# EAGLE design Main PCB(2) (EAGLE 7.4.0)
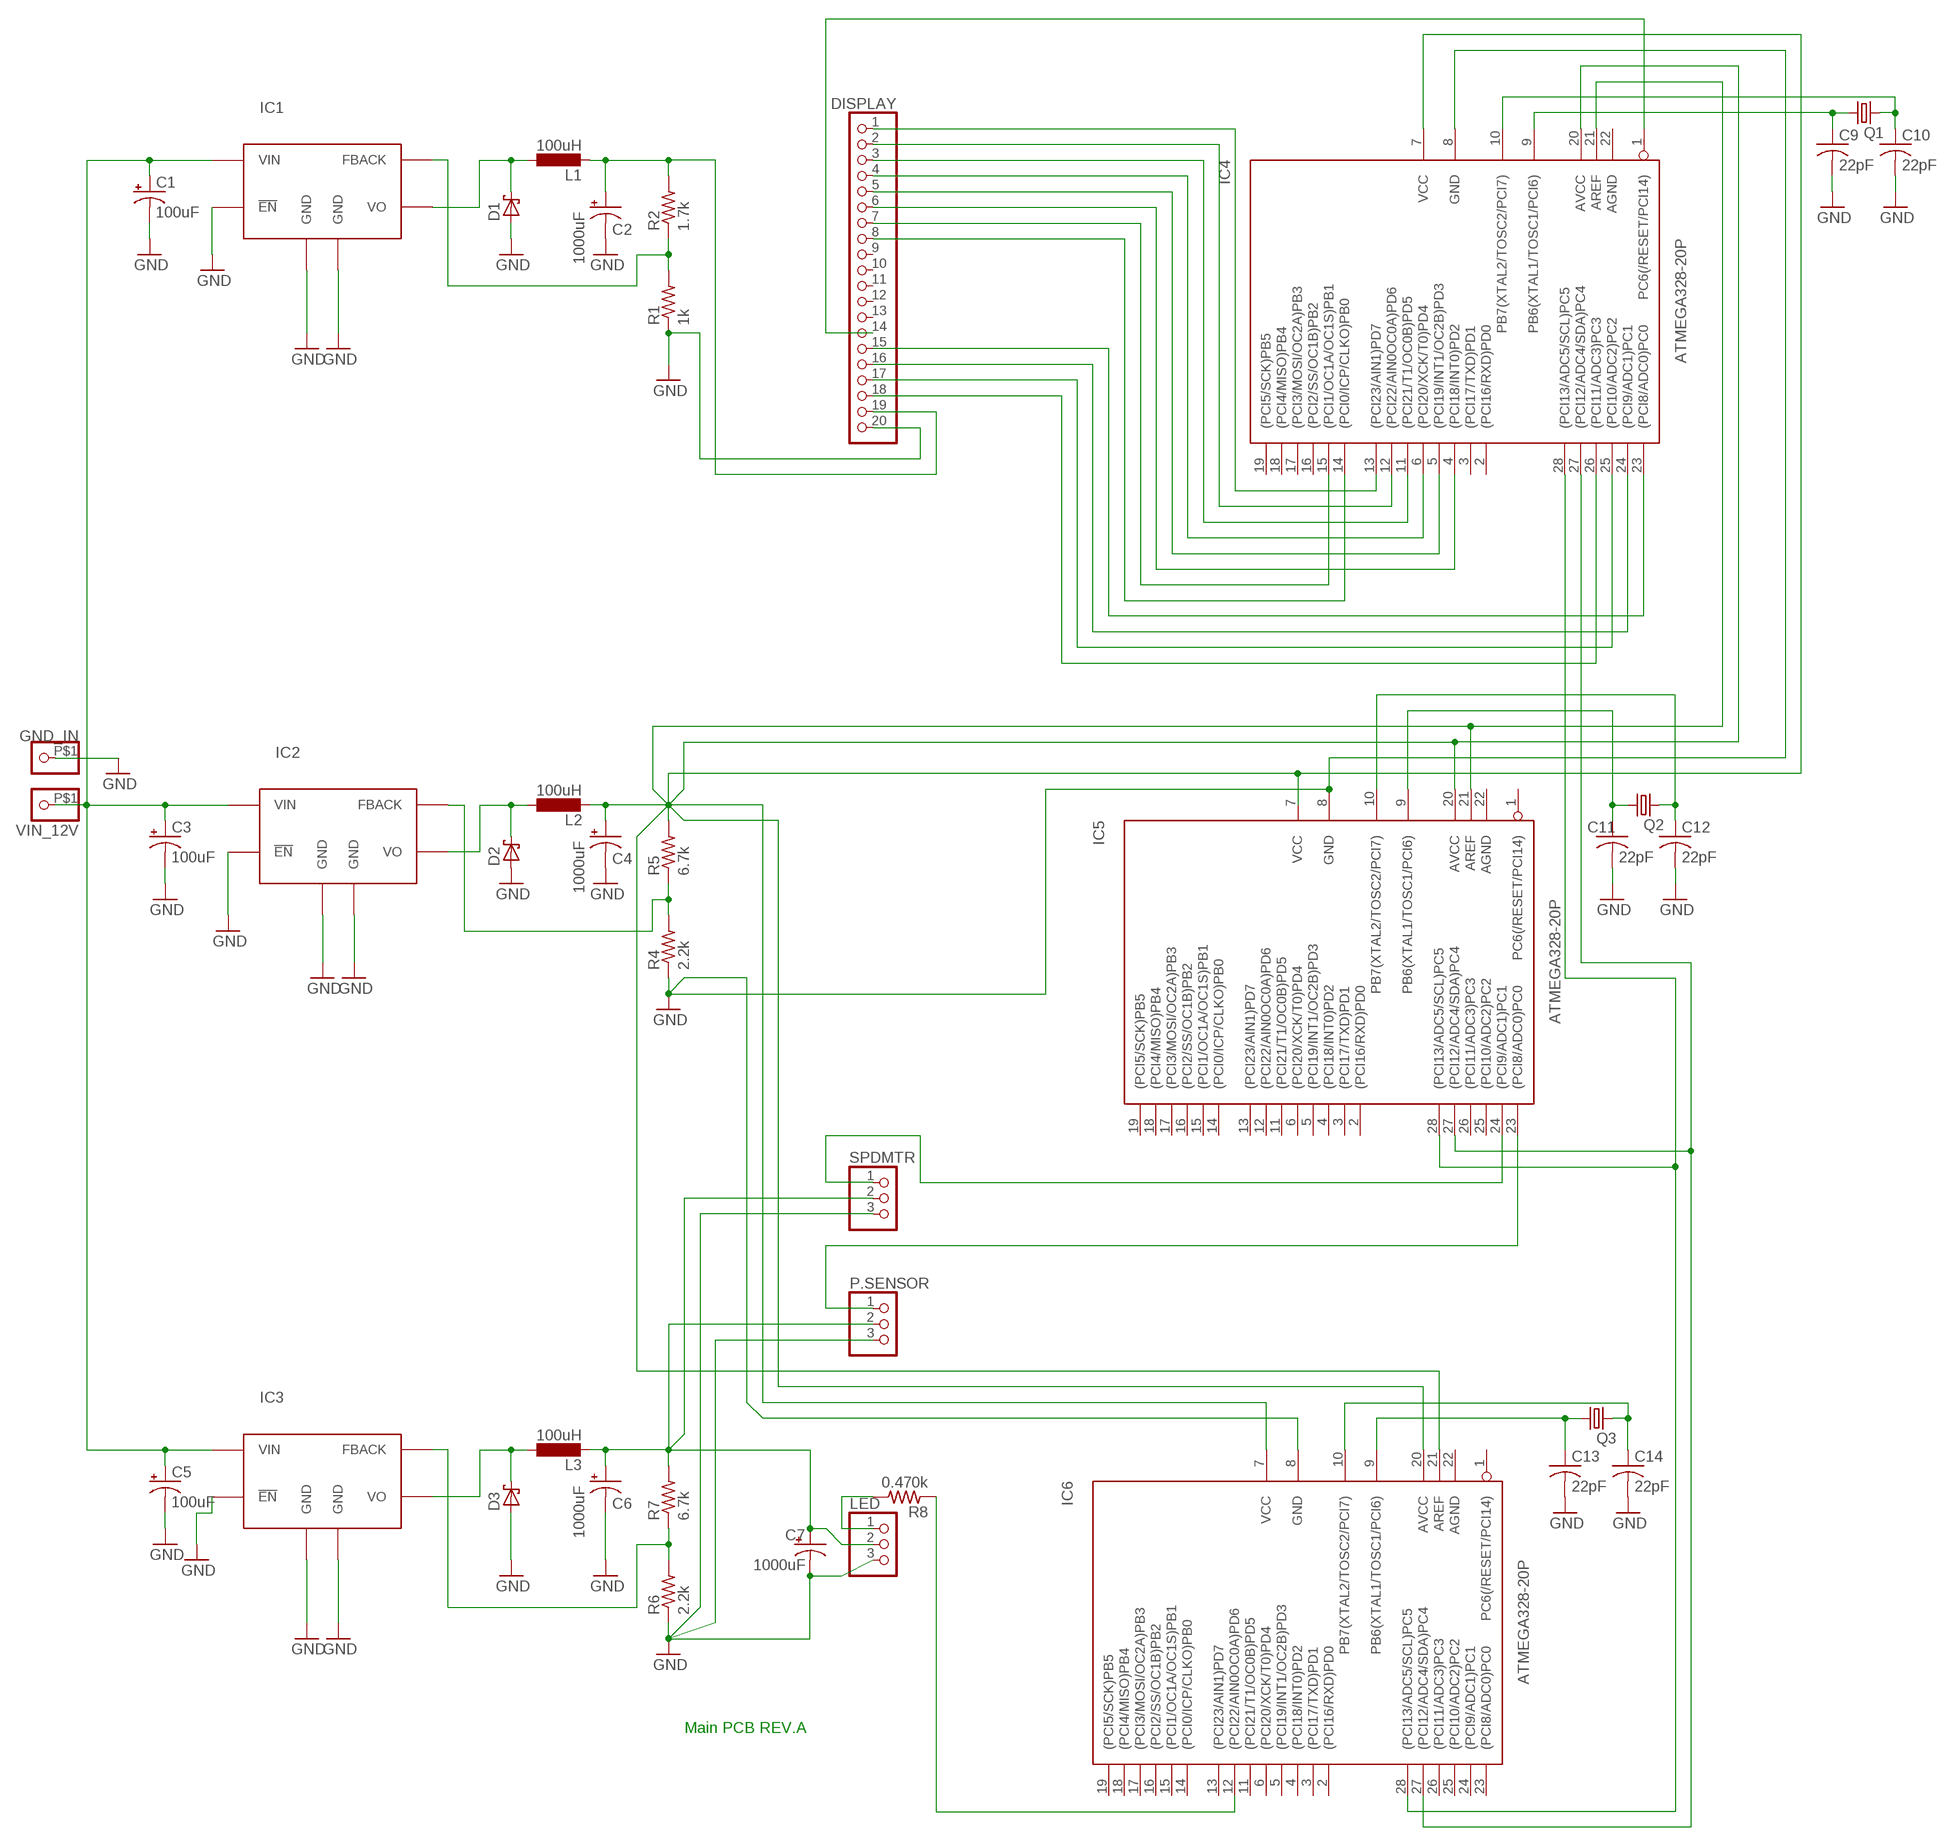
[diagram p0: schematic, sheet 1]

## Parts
C1  100uF  CAP_POLPTH1  [CPOL-RADIAL-100UF-25V]
C2  1000uF  CAP_POLPTH4  [CPOL-RADIAL-1000UF-25V]
C3  100uF  CAP_POLPTH1  [CPOL-RADIAL-100UF-25V]
C4  1000uF  CAP_POLPTH4  [CPOL-RADIAL-1000UF-25V]
C5  100uF  CAP_POLPTH1  [CPOL-RADIAL-100UF-25V]
C6  1000uF  CAP_POLPTH4  [CPOL-RADIAL-1000UF-25V]
C7  1000uF  CAP_POLPTH4  [CPOL-RADIAL-1000UF-25V]
C9  22pF  C-US025-024X044  [C025-024X044]
C10  22pF  C-US025-024X044  [C025-024X044]
C11  22pF  C-US025-024X044  [C025-024X044]
C12  22pF  C-US025-024X044  [C025-024X044]
C13  22pF  C-US025-024X044  [C025-024X044]
C14  22pF  C-US025-024X044  [C025-024X044]
D1  BYV10  [DO41-10]
D2  BYV10  [DO41-10]
D3  BYV10  [DO41-10]
DISPLAY  PINHD-1X20  [1X20]
GND_IN  PINHD-1X1-BIGPOGO  [1X1-BIGPOGO]
IC1  LM2576S  [TO263-5]
IC2  LM2576S  [TO263-5]
IC3  LM2576S  [TO263-5]
IC4  ATMEGA328-20P  [DIL28-3]
IC5  ATMEGA328-20P  [DIL28-3]
IC6  ATMEGA328-20P  [DIL28-3]
L1  100uH  L-EUTJ3-U2  [TJ3-U2]
L2  100uH  L-EUTJ3-U2  [TJ3-U2]
L3  100uH  L-EUTJ3-U2  [TJ3-U2]
LED  PINHD-1X3  [1X03]
P.SENSOR  PINHD-1X3  [1X03]
Q1  CRYSTALTC26V  [TC26V]
Q2  CRYSTALTC26V  [TC26V]
Q3  CRYSTALTC26V  [TC26V]
R1  1k  R-US_0204/5  [0204/5]
R2  1.7k  R-US_0204/5  [0204/5]
R4  2.2k  R-US_0204/5  [0204/5]
R5  6.7k  R-US_0204/5  [0204/5]
R6  2.2k  R-US_0204/5  [0204/5]
R7  6.7k  R-US_0204/5  [0204/5]
R8  0.470k  R-US_0204/5  [0204/5]
SPDMTR  PINHD-1X3  [1X03]
VIN_12V  PINHD-1X1-BIGPOGO  [1X1-BIGPOGO]

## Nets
GND [Supply]: C1.2(-) C2.- C3.2(-) C4.- C5.2(-) C6.- C7.- C9.2 C10.2 C11.2 C12.2 C13.2 C14.2 D1.A D2.A D3.A DISPLAY.20 GND_IN.P$1 IC1.3(GND) IC1.5(!EN) IC1.TAB(GND) IC2.3(GND) IC2.5(!EN) IC2.TAB(GND) IC3.3(GND) IC3.5(!EN) IC3.TAB(GND) IC4.8(GND) IC5.8(GND) IC6.8(GND) LED.3 P.SENSOR.3 R1.1 R4.1 R6.1 SPDMTR.3
LED: IC4.27((PCI12/ADC4/SDA)PC4) IC5.27((PCI12/ADC4/SDA)PC4) IC6.27((PCI12/ADC4/SDA)PC4)
N$1 [Supply]: C1.1(+) C3.1(+) C5.1(+) IC1.1(VIN) IC2.1(VIN) IC3.1(VIN) VIN_12V.P$1
N$2 [Supply]: D1.C IC1.2(VO) L1.1
N$3 [Supply]: D3.C IC3.2(VO) L3.1
N$4: LED.1 R8.2
N$5 [Supply]: IC3.4(FBACK) R6.2 R7.1
N$6: DISPLAY.18 IC4.26((PCI11/ADC3)PC3)
N$7: C12.1 IC5.10(PB7(XTAL2/TOSC2/PCI7)) Q2.2
N$8 [Supply]: IC2.4(FBACK) R4.2 R5.1
N$10: DISPLAY.1 IC4.13((PCI23/AIN1)PD7)
N$11: IC5.24((PCI9/ADC1)PC1) SPDMTR.1
N$12 [Supply]: D2.C IC2.2(VO) L2.1
N$13: IC4.28((PCI13/ADC5/SCL)PC5) IC5.28((PCI13/ADC5/SCL)PC5) IC6.28((PCI13/ADC5/SCL)PC5)
N$14: IC6.12((PCI22/AIN0OC0A)PD6) R8.1
N$15: DISPLAY.2 IC4.12((PCI22/AIN0OC0A)PD6)
N$16: DISPLAY.3 IC4.11((PCI21/T1/OC0B)PD5)
N$17: DISPLAY.4 IC4.6((PCI20/XCK/T0)PD4)
N$18 [Supply]: C4.+ IC4.7(VCC) IC4.20(AVCC) IC4.21(AREF) IC5.20(AVCC) IC5.21(AREF) IC6.7(VCC) IC6.20(AVCC) IC6.21(AREF) L2.2 R5.2
N$19: C11.1 IC5.9(PB6(XTAL1/TOSC1/PCI6)) Q2.1
N$20: C14.1 IC6.10(PB7(XTAL2/TOSC2/PCI7)) Q3.2
N$21: DISPLAY.15 IC4.23((PCI8/ADC0)PC0)
N$22 [Supply]: C2.+ DISPLAY.19 L1.2 R2.2
N$23: IC5.23((PCI8/ADC0)PC0) P.SENSOR.1
N$24: DISPLAY.16 IC4.24((PCI9/ADC1)PC1)
N$25: DISPLAY.17 IC4.25((PCI10/ADC2)PC2)
N$26: DISPLAY.5 IC4.5((PCI19/INT1/OC2B)PD3)
N$27: DISPLAY.6 IC4.4((PCI18/INT0)PD2)
N$28: C13.1 IC6.9(PB6(XTAL1/TOSC1/PCI6)) Q3.1
N$29: DISPLAY.7 IC4.15((PCI1/OC1A/OC1S)PB1)
N$30: DISPLAY.8 IC4.14((PCI0/ICP/CLKO)PB0)
N$31: DISPLAY.14 IC4.1(PC6(/RESET/PCI14))
N$32 [Supply]: C6.+ C7.+ L3.2 LED.2 P.SENSOR.2 R7.2 SPDMTR.2
N$33: C10.1 IC4.10(PB7(XTAL2/TOSC2/PCI7)) Q1.2
N$34: C9.1 IC4.9(PB6(XTAL1/TOSC1/PCI6)) Q1.1
N$38 [Supply]: IC1.4(FBACK) R1.2 R2.1
Unconnected: DISPLAY.9 DISPLAY.10 DISPLAY.11 DISPLAY.12 DISPLAY.13 IC4.2((PCI16/RXD)PD0) IC4.3((PCI17/TXD)PD1) IC4.16((PCI2/SS/OC1B)PB2) IC4.17((PCI3/MOSI/OC2A)PB3) IC4.18((PCI4/MISO)PB4) IC4.19((PCI5/SCK)PB5) IC4.22(AGND) IC5.1(PC6(/RESET/PCI14)) IC5.2((PCI16/RXD)PD0) IC5.3((PCI17/TXD)PD1) IC5.4((PCI18/INT0)PD2) IC5.5((PCI19/INT1/OC2B)PD3) IC5.6((PCI20/XCK/T0)PD4) IC5.7(VCC) IC5.11((PCI21/T1/OC0B)PD5) IC5.12((PCI22/AIN0OC0A)PD6) IC5.13((PCI23/AIN1)PD7) IC5.14((PCI0/ICP/CLKO)PB0) IC5.15((PCI1/OC1A/OC1S)PB1) IC5.16((PCI2/SS/OC1B)PB2) IC5.17((PCI3/MOSI/OC2A)PB3) IC5.18((PCI4/MISO)PB4) IC5.19((PCI5/SCK)PB5) IC5.22(AGND) IC5.25((PCI10/ADC2)PC2) IC5.26((PCI11/ADC3)PC3) IC6.1(PC6(/RESET/PCI14)) IC6.2((PCI16/RXD)PD0) IC6.3((PCI17/TXD)PD1) IC6.4((PCI18/INT0)PD2) IC6.5((PCI19/INT1/OC2B)PD3) IC6.6((PCI20/XCK/T0)PD4) IC6.11((PCI21/T1/OC0B)PD5) IC6.13((PCI23/AIN1)PD7) IC6.14((PCI0/ICP/CLKO)PB0) IC6.15((PCI1/OC1A/OC1S)PB1) IC6.16((PCI2/SS/OC1B)PB2) IC6.17((PCI3/MOSI/OC2A)PB3) IC6.18((PCI4/MISO)PB4) IC6.19((PCI5/SCK)PB5) IC6.22(AGND) IC6.23((PCI8/ADC0)PC0) IC6.24((PCI9/ADC1)PC1) IC6.25((PCI10/ADC2)PC2) IC6.26((PCI11/ADC3)PC3)

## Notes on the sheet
- Main PCB REV.A

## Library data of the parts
C1 C3 C5 = SparkFun-Capacitors:CAP_POL: Capacitor Polarized; MPN: UPW1E101MED; OC_NEWARK: 55K0210
C2 C4 C6 C7 = SparkFun-Capacitors:CAP_POL: Capacitor Polarized; MF: UNITED CHEMI-CON; MPN: EKMG160ELL102MJ16S; OC_NEWARK: 23K3576
C9-C14 = adafruit:C-US: CAPACITOR, American symbol; MPN: MCCC50V220JNPO; OC_NEWARK: 97M5068
D1-D3 = diode:BYV10: DIODE; MPN: 1N5818-E3/54; OC_NEWARK: 78K2605
DISPLAY = adafruit:PINHD-1X20: PIN HEADER; MF: MILL MAX MFG. CORP.; MPN: 310-93-120-41-001; OC_NEWARK: 66F6053
GND_IN VIN_12V = adafruit:PINHD-1X1: Pin header 1x1 for 0.1" spacing; OC_NEWARK: unknown
IC1-IC3 = AWJLEagleLib:LM2576: Texas Instruments LM2576 Simple Switcher
IC4-IC6 = atmega328:ATMEGA328*P: MICROCONTROLLER 32 kBytes FLASH 2 kBytes SRAM 1 kBytes EEPROM USART 8-channel 10 bit ADC; MPN: A000048; OC_NEWARK: 13T9287
L1-L3 = resistor:L-EU: INDUCTOR, European symbol; MPN: RL622-101K-RC; OC_NEWARK: 86K3359
LED P.SENSOR SPDMTR = adafruit:PINHD-1X3: PIN HEADER; OC_NEWARK: unknown
Q1-Q3 = adafruit:CRYSTAL: CRYSTAL; MF: Abracon Corporation; MPN: ABL-20.000MHZ-B2; OC_FARNELL: unknown; OC_NEWARK: 13J1633
R1 R2 R5 R7 R8 = rcl:R-US_: RESISTOR, American symbol; OC_NEWARK: unknown
R4 R6 = rcl:R-US_: RESISTOR, American symbol; MPN: ERJ-2GEJ620X; OC_NEWARK: 53W4174

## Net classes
0 default: width 0.305 mm, drill 0.508 mm, clearance 0.254 mm
1 Supply: width 1.27 mm, drill 0.508 mm, clearance 0.254 mm to class 0, clearance 0.205 mm

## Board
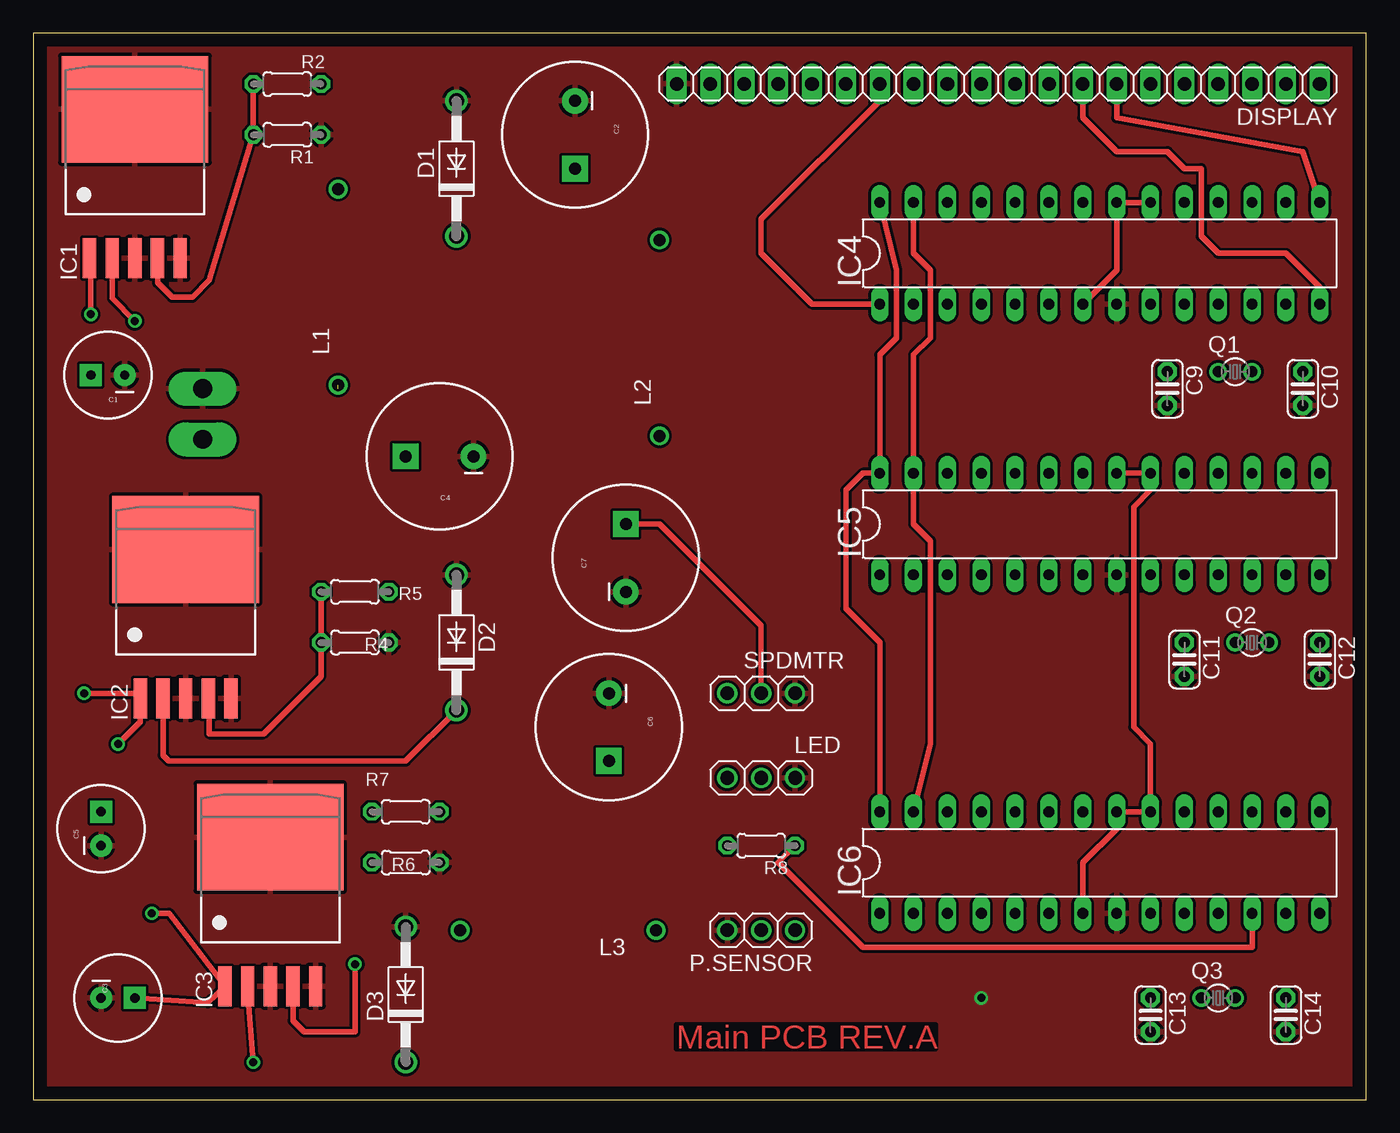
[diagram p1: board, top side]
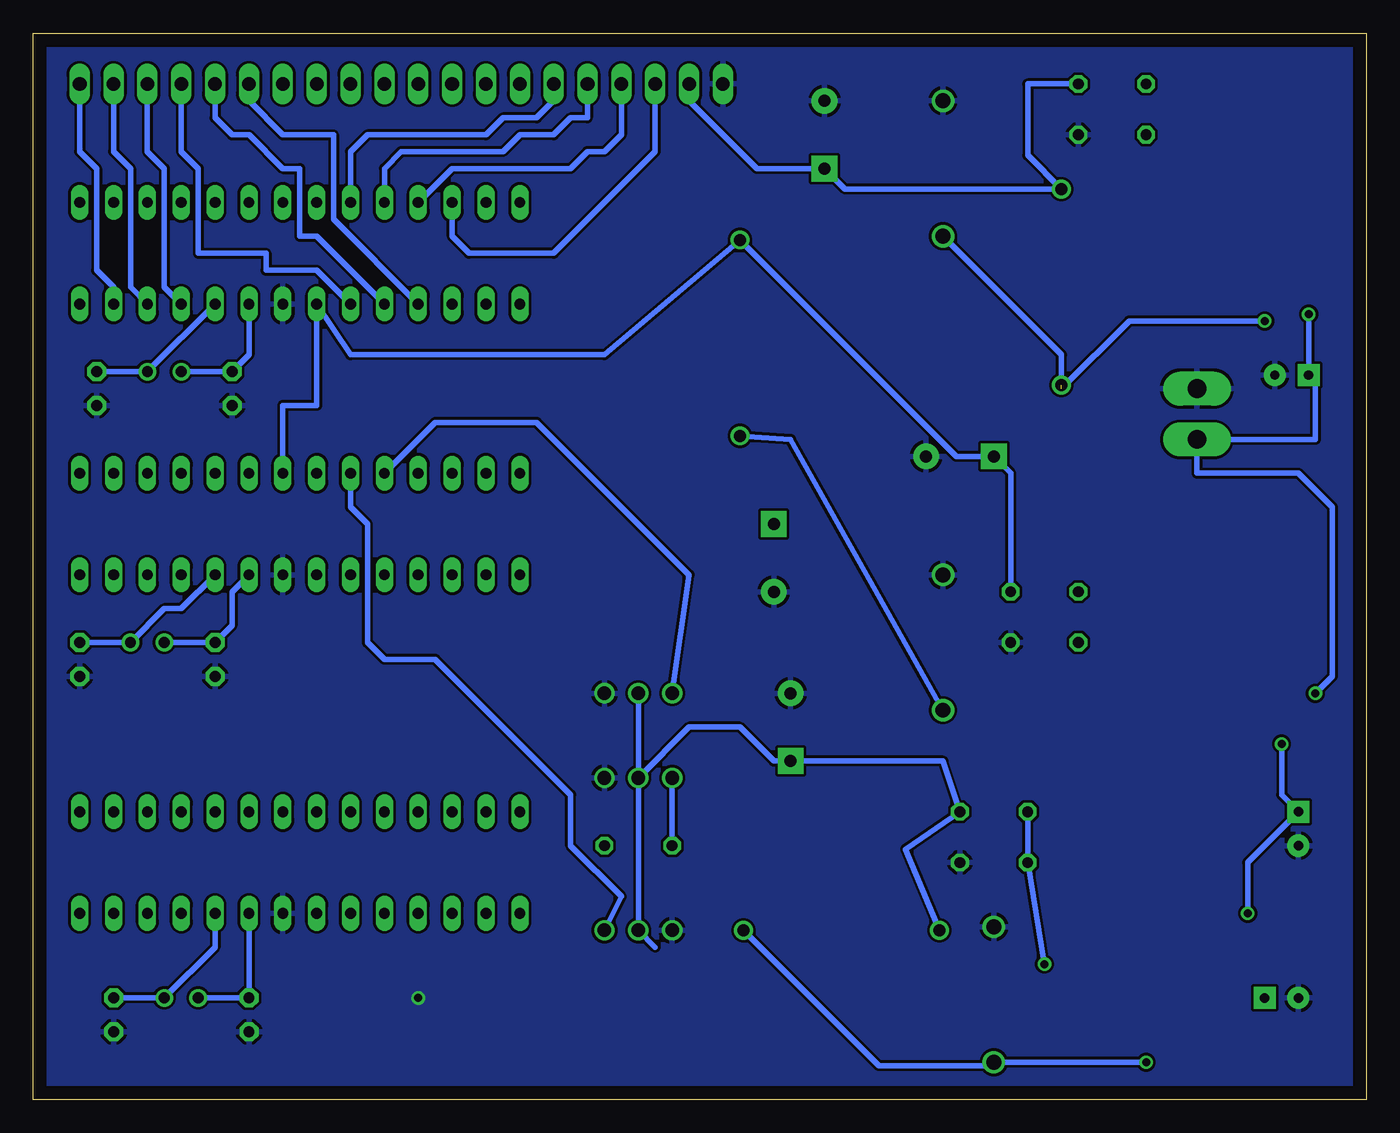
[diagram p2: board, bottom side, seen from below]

Size 100 x 80 mm. Coordinates in mm from the lower left corner, seen from the top.
Outline: 0,0 100,0 100,80 0,80 0,0
Copper layers (1*16): Top 0.035mm / dielectric 1.5mm / Bottom 0.035mm
Design rules "Main PCB(2)": minimum track width 10mil, minimum drill 24mil, track to track 0.205mm, track to pad 0.205mm, pad to pad 0.205mm, via to via 0.205mm, smd to smd 8mil, copper to edge 40mil, drill to drill 8mil, minimum pad ring 10mil, minimum via ring 8mil, stop-mask expansion 4mil, vias tented up to drill 0mil, thermal gap 10mil

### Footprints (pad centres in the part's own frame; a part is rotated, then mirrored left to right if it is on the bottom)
CPOL-RADIAL-100UF-25V = drill 0.7 pad 1.651 square: 1 1.27,0 | drill 0.7 pad 1.651: 2 -1.27,0
CPOL-RADIAL-1000UF-25V = drill 0.9 pad 1.93 square: + 2.54,0 | drill 0.9 pad 1.93: - -2.54,0
C025-024X044 = drill 0.813 pad 1.422 octagon: 1 -1.27,0; 2 1.27,0
DO41-10 = drill 1.118: A 5.08,0; C -5.08,0
1X20 = drill 1.016 long: 1 -24.13,0; 2 -21.59,0; 3 -19.05,0; 4 -16.51,0; 5 -13.97,0; 6 -11.43,0; 7 -8.89,0; 8 -6.35,0; 9 -3.81,0; 10 -1.27,0; 11 1.27,0; 12 3.81,0; 13 6.35,0; 14 8.89,0; 15 11.43,0; 16 13.97,0; 17 16.51,0; 18 19.05,0; 19 21.59,0; 20 24.13,0
1X1-BIGPOGO = drill 1.4 pad 2.54 long: P$1 0,0
TO263-5 = smd 1 x 3: 1 -3.4,-8; 2 -1.7,-8; 3 0,-8; 4 1.7,-8; 5 3.4,-8 | smd 11 x 8: TAB 0,3.175
DIL28-3 = drill 0.813 long: 1 -16.51,-3.81; 2 -13.97,-3.81; 3 -11.43,-3.81; 4 -8.89,-3.81; 5 -6.35,-3.81; 6 -3.81,-3.81; 7 -1.27,-3.81; 8 1.27,-3.81; 9 3.81,-3.81; 10 6.35,-3.81; 11 8.89,-3.81; 12 11.43,-3.81; 13 13.97,-3.81; 14 16.51,-3.81; 15 16.51,3.81; 16 13.97,3.81; 17 11.43,3.81; 18 8.89,3.81; 19 6.35,3.81; 20 3.81,3.81; 21 1.27,3.81; 22 -1.27,3.81; 23 -3.81,3.81; 24 -6.35,3.81; 25 -8.89,3.81; 26 -11.43,3.81; 27 -13.97,3.81; 28 -16.51,3.81
TJ3-U2 = drill 0.9: 1 -7.35,0; 2 7.35,0
1X03 = drill 1.016: 1 -2.54,0; 2 0,0; 3 2.54,0
TC26V = drill 0.813: 1 -1.27,0; 2 1.27,0
0204/5 = drill 0.813 octagon: 1 -2.54,0; 2 2.54,0

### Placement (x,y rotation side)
C1  5.59,54.36 180 top
C2  40.64,72.39 270 top
C3  6.35,7.62 0 top
C4  30.48,48.26 180 top
C5  5.08,20.32 90 top
C6  43.18,27.94 270 top
C7  44.45,40.64 90 top
C9  85.09,53.34 270 top
C10  95.25,53.34 270 top
C11  86.36,33.02 270 top
C12  96.52,33.02 270 top
C13  83.82,6.35 270 top
C14  93.98,6.35 270 top
D1  31.75,69.85 90 top
D2  31.75,34.29 90 top
D3  27.94,7.87 90 top
DISPLAY  72.39,76.2 180 top
GND_IN  12.7,53.34 0 top
IC1  7.62,71.12 0 top
IC2  11.43,38.1 0 top
IC3  17.78,16.51 0 top
IC4  80.01,63.5 0 top
IC5  80.01,43.18 0 top
IC6  80.01,17.78 0 top
L1  22.86,60.96 90 top
L2  46.99,57.15 90 top
L3  39.37,12.7 180 top
LED  54.61,24.13 0 top
P.SENSOR  54.61,12.7 180 top
Q1  90.17,54.61 0 top
Q2  91.44,34.29 0 top
Q3  88.9,7.62 0 top
R1  19.05,72.39 180 top
R2  19.05,76.2 0 top
R4  24.13,34.29 180 top
R5  24.13,38.1 0 top
R6  27.94,17.78 180 top
R7  27.94,21.59 0 top
R8  54.61,19.05 180 top
SPDMTR  54.61,30.48 0 top
VIN_12V  12.7,49.53 0 top

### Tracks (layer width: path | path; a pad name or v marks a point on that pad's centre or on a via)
GND  (via drill 0.6)
  other vias: 71.12,7.62
  pour Top: -1.27,81.28 -1.27,-1.27 101.6,-1.27 101.6,81.28
  pour Bottom: -2.54,82.55 -2.54,-2.54 102.87,-2.54 102.87,-1.27 102.87,82.55
LED
  Top 0.406: IC4.27 66.04,63.5 67.31,62.23 67.31,57.15 66.04,55.88 IC5.27 66.04,43.18 67.31,41.91 67.31,26.67 IC6.27
N$1  (via drill 0.6)
  Top 0.406: IC1.1 4.32,63.12 v4.32,58.93 | v3.81,30.48 7.65,30.48 IC2.1 8.03,28.35 v6.35,26.67 | v8.89,13.97 10.19,13.97 IC3.1 13.08,7.24 C3.1
  Bottom 0.406: v4.32,58.93 C1.1 3.81,54.36 3.81,49.53 VIN_12V.P$1 12.7,46.99 5.08,46.99 2.54,44.45 2.54,31.75 v3.81,30.48 | v6.35,26.67 6.35,22.86 C5.1 8.89,17.78 v8.89,13.97
N$2  (via drill 0.6)  (1 unrouted)
  Top 0.406: IC1.2 5.92,60.12 v7.62,58.42
  Bottom 0.406: v7.62,58.42 17.78,58.42 22.86,53.34 | L1.1 22.86,55.88 D1.C
N$3  (via drill 0.6)
  Top 0.406: IC3.2 16.08,8.05 v16.51,2.79
  Bottom 0.406: v16.51,2.79 D3.C 27.94,2.54 36.56,2.54 L3.1
N$4
  Bottom 0.406: LED.1 R8.2
N$5  (via drill 0.6)
  Top 0.406: IC3.4 19.48,5.92 20.32,5.08 24.13,5.08 v24.13,10.16
  Bottom 0.406: v24.13,10.16 R6.2 R7.1
N$6
  Bottom 0.406: DISPLAY.18 53.34,71.12 60.96,63.5 67.31,63.5 68.58,64.77 IC4.26
N$7
  Bottom 0.406: IC5.10 88.9,36.83 90.17,36.83 Q2.2 C12.1
N$8
  Top 0.406: IC2.4 13.21,30.1 13.21,27.43 17.27,27.43 21.59,31.75 R4.2 R5.1
N$10
  Bottom 0.406: DISPLAY.1 96.52,71.12 95.25,69.85 95.25,62.23 93.98,60.96 IC4.13
N$11
  Bottom 0.406: SPDMTR.1 50.8,39.37 62.23,50.8 69.85,50.8 IC5.24
N$12
  Top 0.406: IC2.2 9.73,25.83 10.16,25.4 27.94,25.4 D2.C
  Bottom 0.406: D2.C 43.18,49.53 L2.1
N$13
  Top 0.406: IC6.28 63.5,34.29 60.96,36.83 60.96,45.72 62.23,46.99 IC5.28 63.5,55.88 64.77,57.15 64.77,62.23 IC4.28
N$14
  Top 0.406: R8.1 55.88,17.78 62.23,11.43 91.44,11.43 IC6.12
N$15
  Bottom 0.406: DISPLAY.2 93.98,71.12 92.71,69.85 92.71,60.96 IC4.12
N$16
  Bottom 0.406: DISPLAY.3 91.44,71.12 90.17,69.85 90.17,60.96 IC4.11
N$17
  Bottom 0.406: DISPLAY.4 88.9,71.12 87.63,69.85 87.63,63.5 82.55,63.5 82.55,62.23 78.74,62.23 IC4.6
N$18
  Top 0.406: IC5.21 IC5.20 83.82,45.72 82.55,44.45 82.55,27.94 83.82,26.67 IC6.20 IC6.21 81.28,20.32 78.74,17.78 IC6.7 | IC4.20 IC4.21 81.28,62.23 IC4.7
  Bottom 0.406: IC5.21 81.28,52.07 78.74,52.07 IC4.7 76.2,55.88 57.15,55.88 L2.2 30.75,48.26 C4.+ 26.67,46.99 R5.2
N$19
  Bottom 0.406: IC5.9 85.09,38.1 85.09,35.56 C11.1 Q2.1
N$20
  Bottom 0.406: IC6.10 86.36,11.43 Q3.2 C14.1
N$21
  Bottom 0.406: DISPLAY.15 60.96,74.93 62.23,73.66 64.77,73.66 66.04,72.39 74.93,72.39 76.2,71.12 IC4.23
N$22
  Bottom 0.406: DISPLAY.19 50.8,74.93 45.72,69.85 C2.+ 39.1,68.31 L1.2 25.4,70.85 25.4,76.2 R2.2
N$23
  Bottom 0.406: P.SENSOR.1 55.88,15.24 59.69,19.05 59.69,22.86 69.85,33.02 73.66,33.02 74.93,34.29 74.93,43.18 76.2,44.45 IC5.23
N$24
  Bottom 0.406: DISPLAY.16 58.42,73.66 59.69,73.66 60.96,72.39 63.5,72.39 64.77,71.12 72.39,71.12 73.66,69.85 IC4.24
N$25
  Bottom 0.406: DISPLAY.17 55.88,72.39 57.15,71.12 58.42,71.12 59.69,69.85 68.58,69.85 IC4.25
N$26
  Bottom 0.406: DISPLAY.5 86.36,73.66 85.09,72.39 83.82,72.39 81.28,69.85 80.01,69.85 80.01,64.77 78.74,64.77 IC4.5
N$27
  Bottom 0.406: DISPLAY.6 83.82,74.93 81.28,72.39 77.47,72.39 77.47,66.04 IC4.4
N$28
  Bottom 0.406: IC6.9 C13.1 Q3.1
N$29
  Top 0.406: DISPLAY.7 81.28,73.66 95.25,71.12 IC4.15
N$30
  Top 0.406: DISPLAY.8 78.74,73.66 81.28,71.12 85.09,71.12 86.36,69.85 87.63,69.85 87.63,64.77 88.9,63.5 93.98,63.5 96.52,60.96 IC4.14
N$31
  Top 0.406: DISPLAY.14 63.5,74.93 54.61,66.04 54.61,63.5 58.42,59.69 IC4.1
N$32
  Top 0.406: C7.+ 46.99,43.18 54.61,35.56 SPDMTR.2
  Bottom 0.406: SPDMTR.2 LED.2 | LED.2 P.SENSOR.2 53.34,11.43 | L3.2 34.56,18.78 R7.2 31.75,25.4 C6.+ 44.45,25.4 46.99,27.94 50.8,27.94 LED.2
N$33
  Bottom 0.406: IC4.10 Q1.2 C10.1
N$34
  Bottom 0.406: IC4.9 83.82,55.88 C9.1 Q1.1
N$38
  Top 0.406: IC1.4 9.32,61.29 10.41,60.2 11.94,60.2 13.21,61.47 R1.2 R2.1

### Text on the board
Top: Main PCB REV.A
